(* Logix 5000 AddOnInstructionDefinition export Banner_Q2X_Param_v4; software revision 33.00; part 2 of 3 *)
(* tags used below, declared in another part *)
   Q2X : Banner_Q2X_v4;
   Port_Data : Banner_IOL_Port_v4;
   Port : DINT;
   Local_Control : DINT;
   Command_Being_Processed : BOOL;
   Update_Archive : BOOL;
   Index_Write_Inprocess : INT;
   Index_Write_Control : INT;
   Inprocess_Index : DINT;
(* Banner_Q2X_Param_v4, continued *)

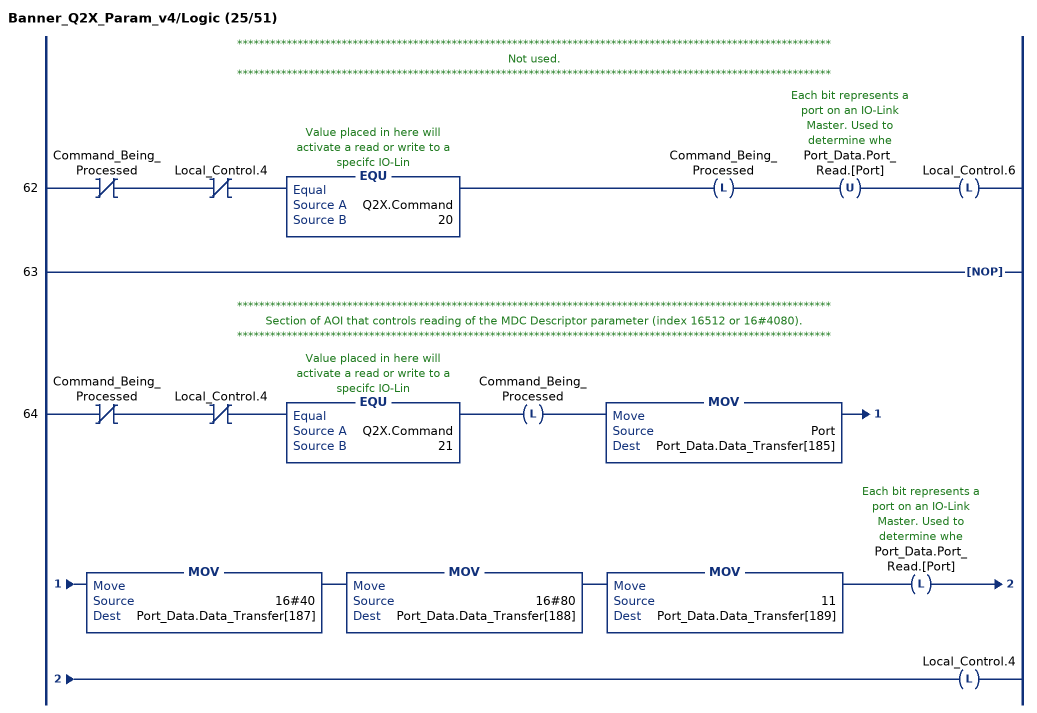
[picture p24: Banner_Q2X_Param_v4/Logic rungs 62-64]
   // ************************************************************************************************************
   // Not used.
   // ************************************************************************************************************
   62: XIO(Command_Being_Processed)XIO(Local_Control.4)EQU(Q2X.Command,20)OTL(Command_Being_Processed)OTU(Port_Data.Port_Read.[Port])OTL(Local_Control.6);
   63: NOP();
   // ************************************************************************************************************
   // Section of AOI that controls reading of the MDC Descriptor parameter (index 16512 or 16#4080).
   // ************************************************************************************************************
   64: XIO(Command_Being_Processed)XIO(Local_Control.4)EQU(Q2X.Command,21)OTL(Command_Being_Processed)MOV(Port,Port_Data.Data_Transfer[185])MOV(16#40,Port_Data.Data_Transfer[187])MOV(16#80,Port_Data.Data_Transfer[188])MOV(11,Port_Data.Data_Transfer[189])OTL(Port_Data.Port_Read.[Port])OTL(Local_Control.4);
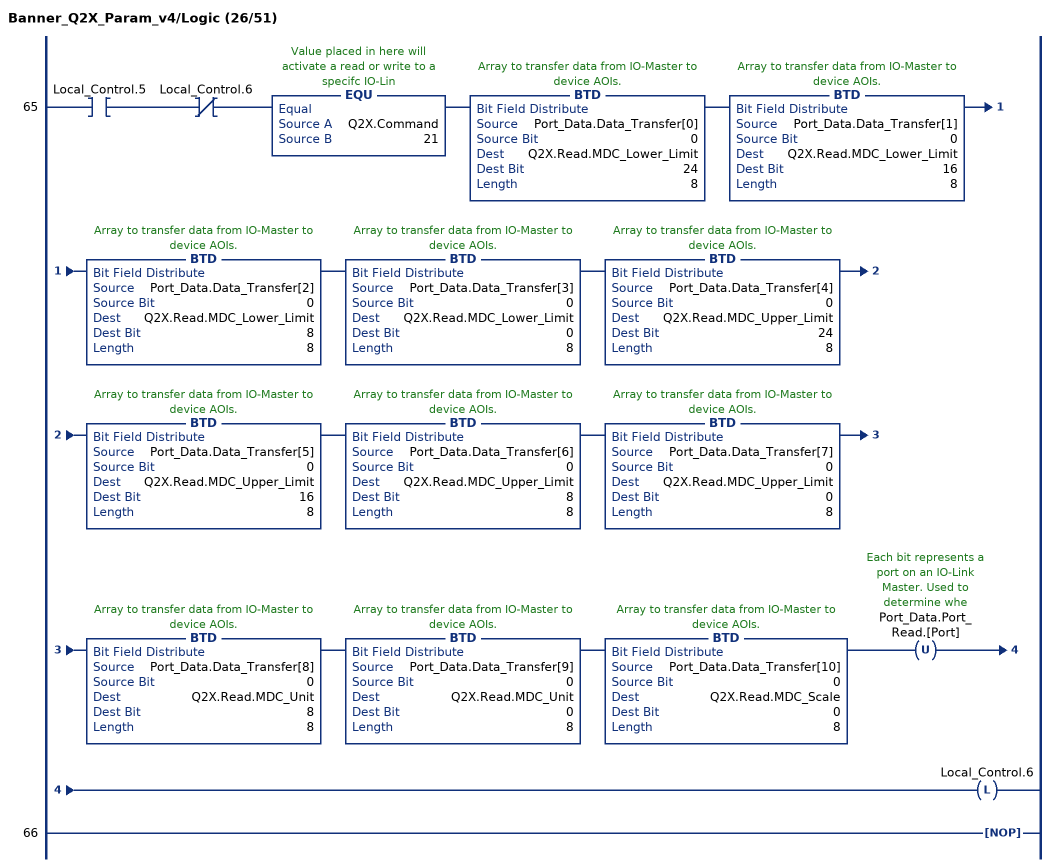
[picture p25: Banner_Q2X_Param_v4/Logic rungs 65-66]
   65: XIC(Local_Control.5)XIO(Local_Control.6)EQU(Q2X.Command,21)BTD(Port_Data.Data_Transfer[0],0,Q2X.Read.MDC_Lower_Limit,24,8)BTD(Port_Data.Data_Transfer[1],0,Q2X.Read.MDC_Lower_Limit,16,8)BTD(Port_Data.Data_Transfer[2],0,Q2X.Read.MDC_Lower_Limit,8,8)BTD(Port_Data.Data_Transfer[3],0,Q2X.Read.MDC_Lower_Limit,0,8)BTD(Port_Data.Data_Transfer[4],0,Q2X.Read.MDC_Upper_Limit,24,8)BTD(Port_Data.Data_Transfer[5],0,Q2X.Read.MDC_Upper_Limit,16,8)BTD(Port_Data.Data_Transfer[6],0,Q2X.Read.MDC_Upper_Limit,8,8)BTD(Port_Data.Data_Transfer[7],0,Q2X.Read.MDC_Upper_Limit,0,8)BTD(Port_Data.Data_Transfer[8],0,Q2X.Read.MDC_Unit,8,8)BTD(Port_Data.Data_Transfer[9],0,Q2X.Read.MDC_Unit,0,8)BTD(Port_Data.Data_Transfer[10],0,Q2X.Read.MDC_Scale,0,8)OTU(Port_Data.Port_Read.[Port])OTL(Local_Control.6);
   66: NOP();
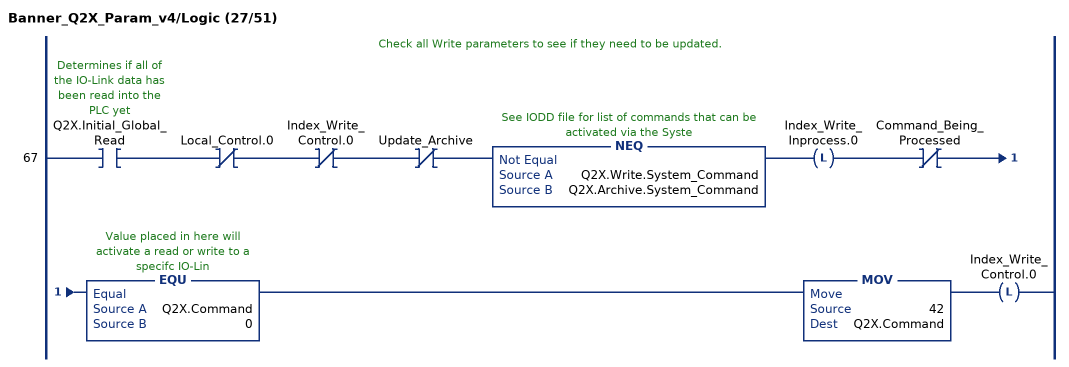
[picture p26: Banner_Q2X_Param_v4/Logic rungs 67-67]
   // Check all Write parameters to see if they need to be updated.
   67: XIC(Q2X.Initial_Global_Read)XIO(Local_Control.0)XIO(Index_Write_Control.0)XIO(Update_Archive)NEQ(Q2X.Write.System_Command,Q2X.Archive.System_Command)OTL(Index_Write_Inprocess.0)XIO(Command_Being_Processed)EQU(Q2X.Command,0)MOV(42,Q2X.Command)OTL(Index_Write_Control.0);
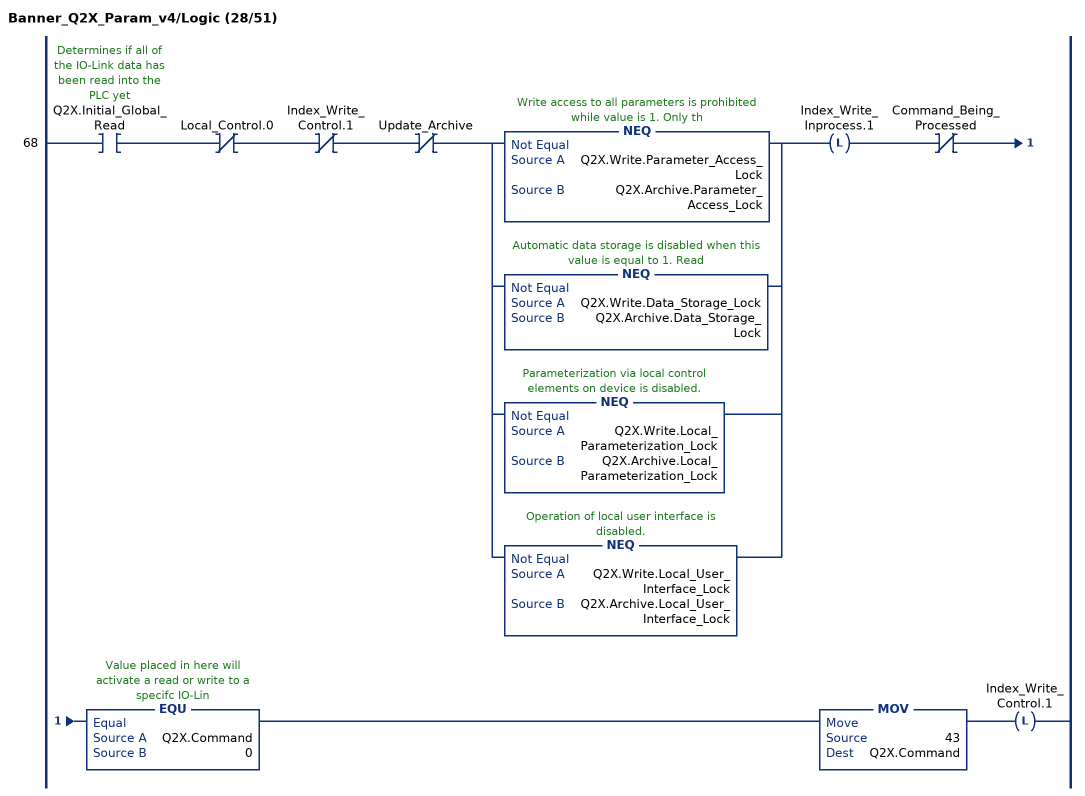
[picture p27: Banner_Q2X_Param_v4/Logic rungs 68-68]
   68: XIC(Q2X.Initial_Global_Read)XIO(Local_Control.0)XIO(Index_Write_Control.1)XIO(Update_Archive)[NEQ(Q2X.Write.Parameter_Access_Lock,Q2X.Archive.Parameter_Access_Lock) ,NEQ(Q2X.Write.Data_Storage_Lock,Q2X.Archive.Data_Storage_Lock) ,NEQ(Q2X.Write.Local_Parameterization_Lock,Q2X.Archive.Local_Parameterization_Lock) ,NEQ(Q2X.Write.Local_User_Interface_Lock,Q2X.Archive.Local_User_Interface_Lock) ]OTL(Index_Write_Inprocess.1)XIO(Command_Being_Processed)EQU(Q2X.Command,0)MOV(43,Q2X.Command)OTL(Index_Write_Control.1);
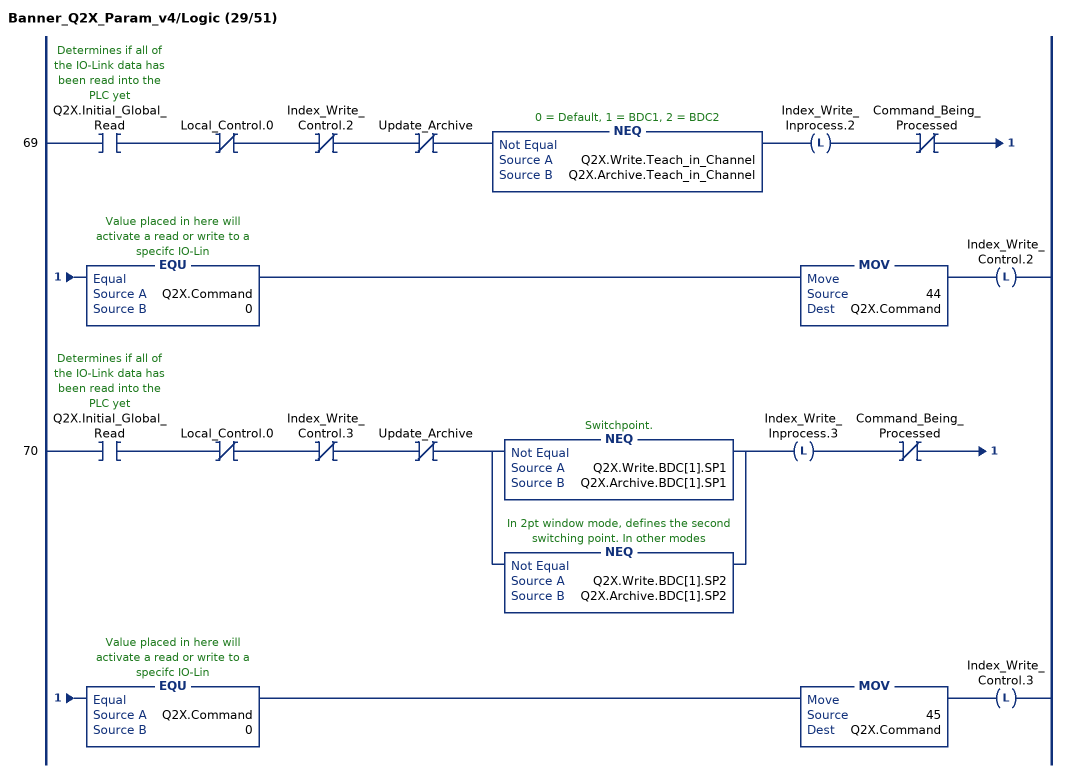
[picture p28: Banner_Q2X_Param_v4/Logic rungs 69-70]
   69: XIC(Q2X.Initial_Global_Read)XIO(Local_Control.0)XIO(Index_Write_Control.2)XIO(Update_Archive)NEQ(Q2X.Write.Teach_in_Channel,Q2X.Archive.Teach_in_Channel)OTL(Index_Write_Inprocess.2)XIO(Command_Being_Processed)EQU(Q2X.Command,0)MOV(44,Q2X.Command)OTL(Index_Write_Control.2);
   70: XIC(Q2X.Initial_Global_Read)XIO(Local_Control.0)XIO(Index_Write_Control.3)XIO(Update_Archive)[NEQ(Q2X.Write.BDC[1].SP1,Q2X.Archive.BDC[1].SP1) ,NEQ(Q2X.Write.BDC[1].SP2,Q2X.Archive.BDC[1].SP2) ]OTL(Index_Write_Inprocess.3)XIO(Command_Being_Processed)EQU(Q2X.Command,0)MOV(45,Q2X.Command)OTL(Index_Write_Control.3);
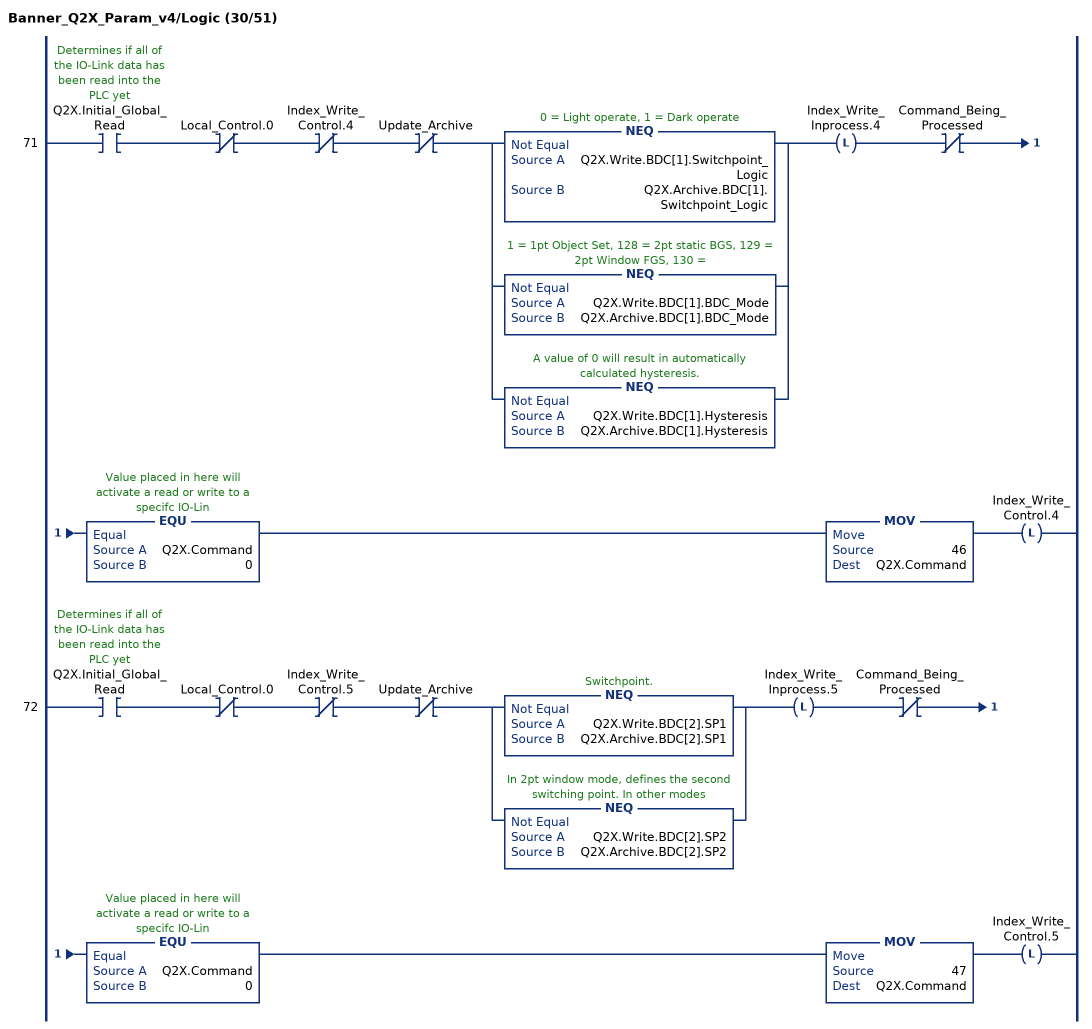
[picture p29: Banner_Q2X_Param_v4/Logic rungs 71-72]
   71: XIC(Q2X.Initial_Global_Read)XIO(Local_Control.0)XIO(Index_Write_Control.4)XIO(Update_Archive)[NEQ(Q2X.Write.BDC[1].Switchpoint_Logic,Q2X.Archive.BDC[1].Switchpoint_Logic) ,NEQ(Q2X.Write.BDC[1].BDC_Mode,Q2X.Archive.BDC[1].BDC_Mode) ,NEQ(Q2X.Write.BDC[1].Hysteresis,Q2X.Archive.BDC[1].Hysteresis) ]OTL(Index_Write_Inprocess.4)XIO(Command_Being_Processed)EQU(Q2X.Command,0)MOV(46,Q2X.Command)OTL(Index_Write_Control.4);
   72: XIC(Q2X.Initial_Global_Read)XIO(Local_Control.0)XIO(Index_Write_Control.5)XIO(Update_Archive)[NEQ(Q2X.Write.BDC[2].SP1,Q2X.Archive.BDC[2].SP1) ,NEQ(Q2X.Write.BDC[2].SP2,Q2X.Archive.BDC[2].SP2) ]OTL(Index_Write_Inprocess.5)XIO(Command_Being_Processed)EQU(Q2X.Command,0)MOV(47,Q2X.Command)OTL(Index_Write_Control.5);
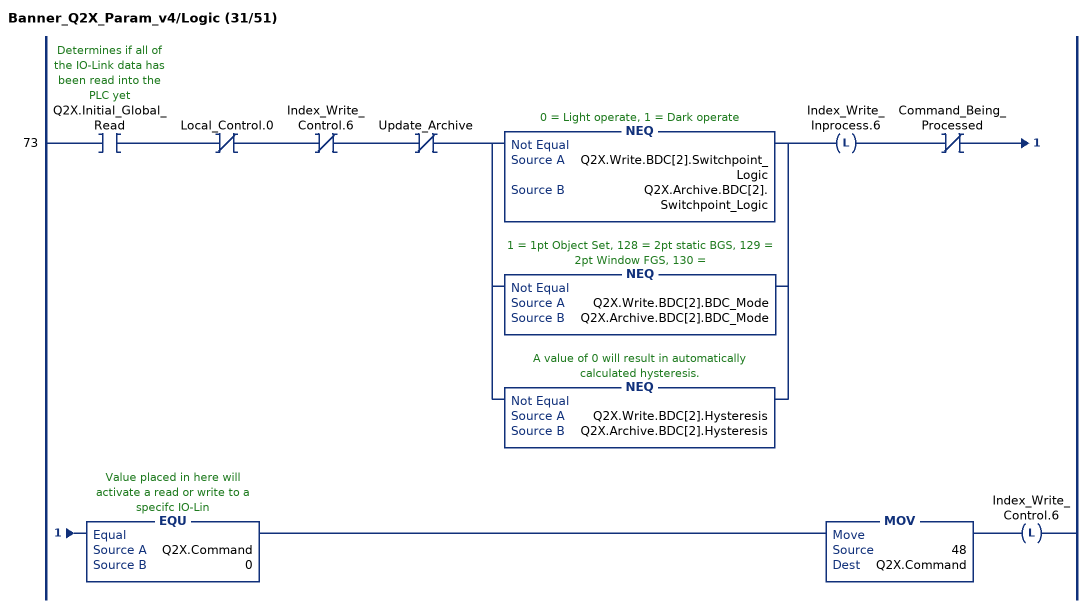
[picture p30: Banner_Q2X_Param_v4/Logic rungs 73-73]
   73: XIC(Q2X.Initial_Global_Read)XIO(Local_Control.0)XIO(Index_Write_Control.6)XIO(Update_Archive)[NEQ(Q2X.Write.BDC[2].Switchpoint_Logic,Q2X.Archive.BDC[2].Switchpoint_Logic) ,NEQ(Q2X.Write.BDC[2].BDC_Mode,Q2X.Archive.BDC[2].BDC_Mode) ,NEQ(Q2X.Write.BDC[2].Hysteresis,Q2X.Archive.BDC[2].Hysteresis) ]OTL(Index_Write_Inprocess.6)XIO(Command_Being_Processed)EQU(Q2X.Command,0)MOV(48,Q2X.Command)OTL(Index_Write_Control.6);
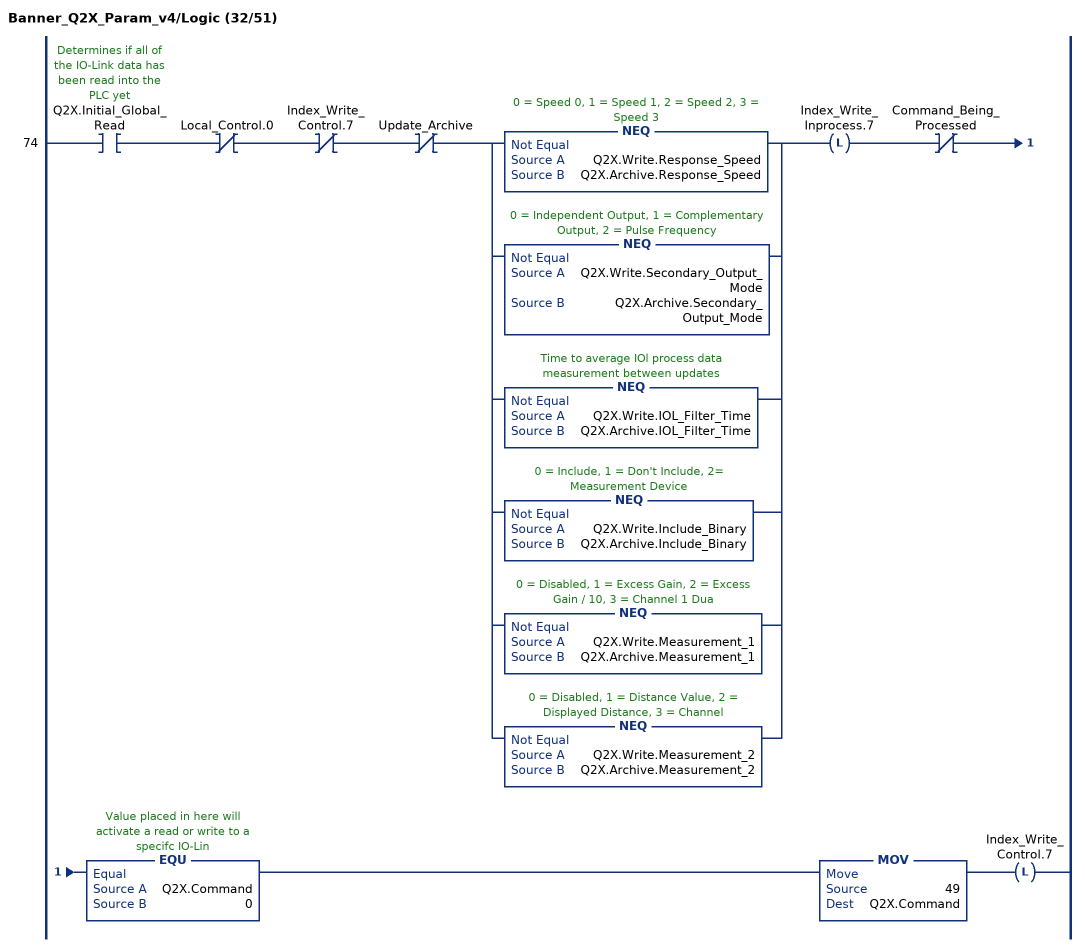
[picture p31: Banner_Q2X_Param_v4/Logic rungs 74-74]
   74: XIC(Q2X.Initial_Global_Read)XIO(Local_Control.0)XIO(Index_Write_Control.7)XIO(Update_Archive)[NEQ(Q2X.Write.Response_Speed,Q2X.Archive.Response_Speed) ,NEQ(Q2X.Write.Secondary_Output_Mode,Q2X.Archive.Secondary_Output_Mode) ,NEQ(Q2X.Write.IOL_Filter_Time,Q2X.Archive.IOL_Filter_Time) ,NEQ(Q2X.Write.Include_Binary,Q2X.Archive.Include_Binary) ,NEQ(Q2X.Write.Measurement_1,Q2X.Archive.Measurement_1) ,NEQ(Q2X.Write.Measurement_2,Q2X.Archive.Measurement_2) ]OTL(Index_Write_Inprocess.7)XIO(Command_Being_Processed)EQU(Q2X.Command,0)MOV(49,Q2X.Command)OTL(Index_Write_Control.7);
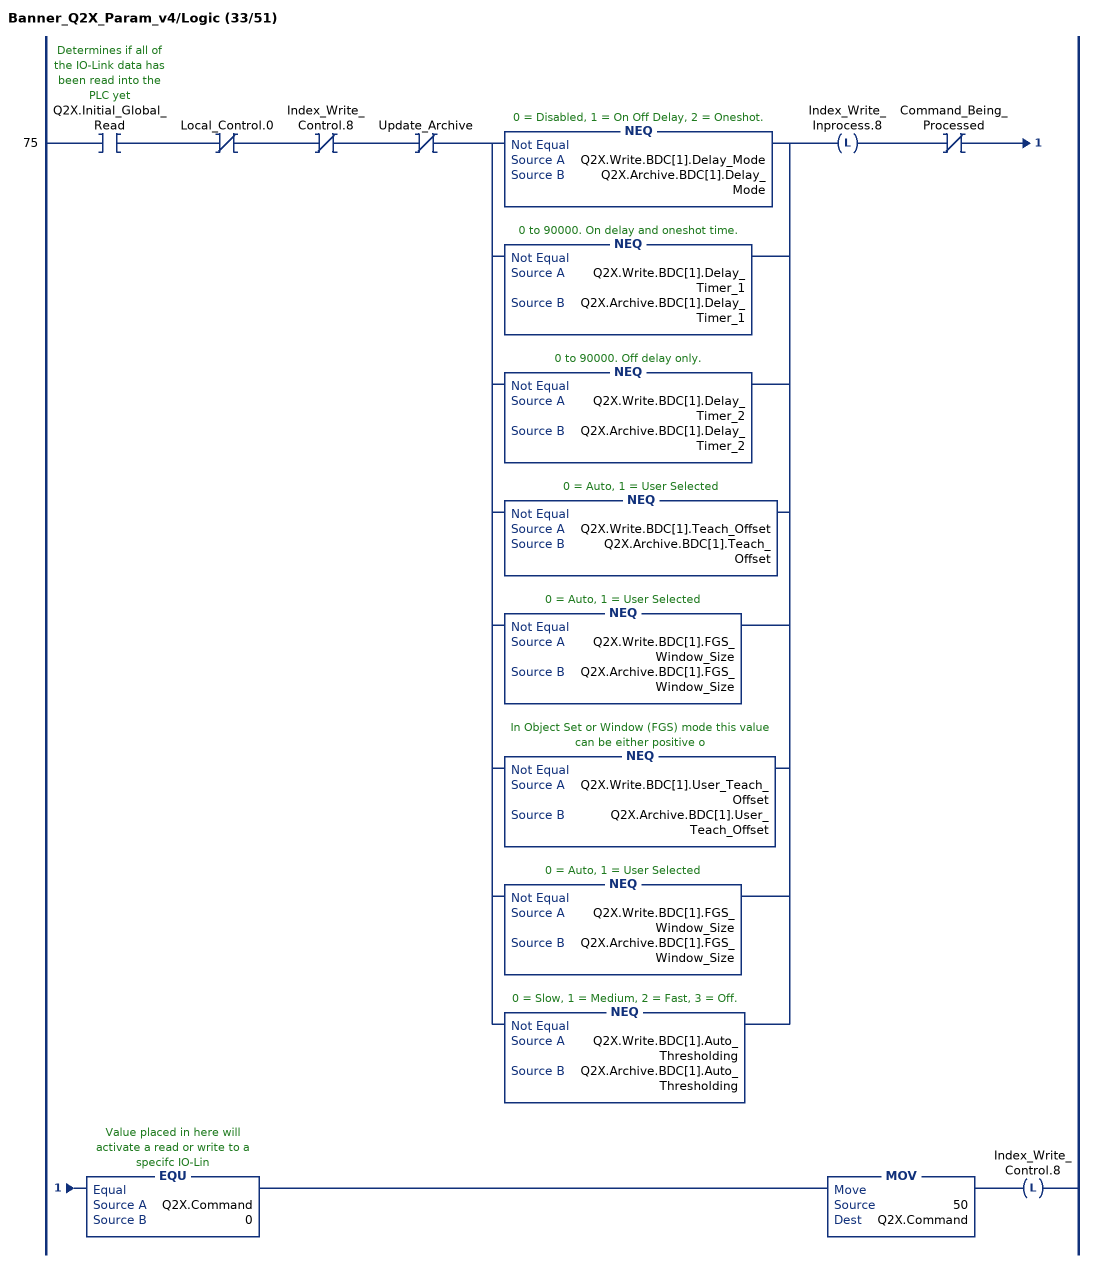
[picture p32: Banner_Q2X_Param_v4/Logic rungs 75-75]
   75: XIC(Q2X.Initial_Global_Read)XIO(Local_Control.0)XIO(Index_Write_Control.8)XIO(Update_Archive)[NEQ(Q2X.Write.BDC[1].Delay_Mode,Q2X.Archive.BDC[1].Delay_Mode) ,NEQ(Q2X.Write.BDC[1].Delay_Timer_1,Q2X.Archive.BDC[1].Delay_Timer_1) ,NEQ(Q2X.Write.BDC[1].Delay_Timer_2,Q2X.Archive.BDC[1].Delay_Timer_2) ,NEQ(Q2X.Write.BDC[1].Teach_Offset,Q2X.Archive.BDC[1].Teach_Offset) ,NEQ(Q2X.Write.BDC[1].FGS_Window_Size,Q2X.Archive.BDC[1].FGS_Window_Size) ,NEQ(Q2X.Write.BDC[1].User_Teach_Offset,Q2X.Archive.BDC[1].User_Teach_Offset) ,NEQ(Q2X.Write.BDC[1].FGS_Window_Size,Q2X.Archive.BDC[1].FGS_Window_Size) ,NEQ(Q2X.Write.BDC[1].Auto_Thresholding,Q2X.Archive.BDC[1].Auto_Thresholding) ]OTL(Index_Write_Inprocess.8)XIO(Command_Being_Processed)EQU(Q2X.Command,0)MOV(50,Q2X.Command)OTL(Index_Write_Control.8);
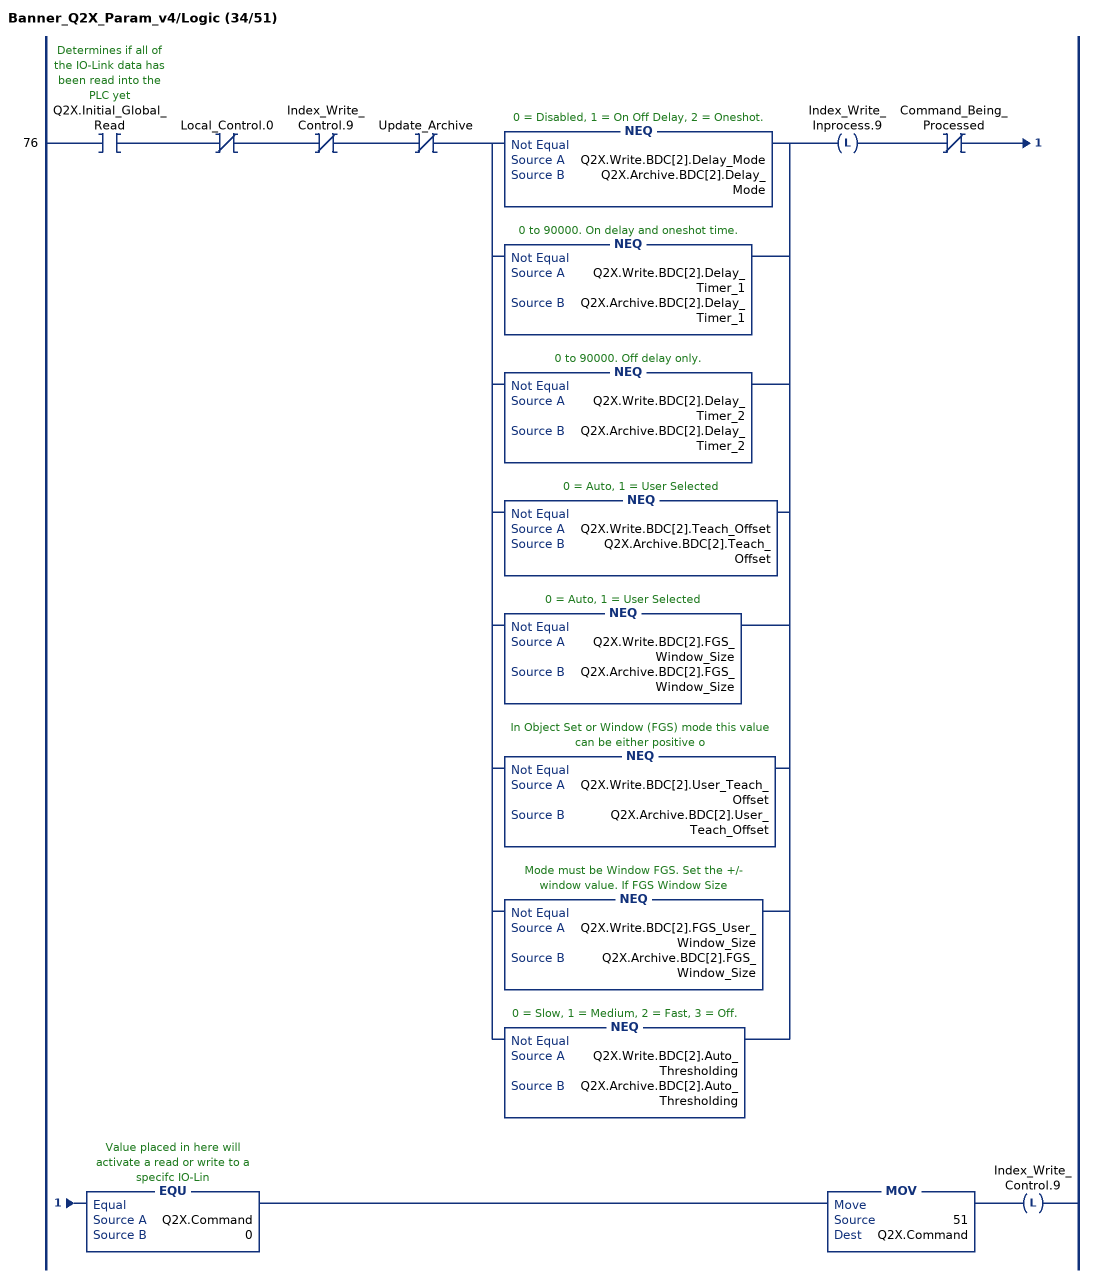
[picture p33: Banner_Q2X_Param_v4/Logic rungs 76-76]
   76: XIC(Q2X.Initial_Global_Read)XIO(Local_Control.0)XIO(Index_Write_Control.9)XIO(Update_Archive)[NEQ(Q2X.Write.BDC[2].Delay_Mode,Q2X.Archive.BDC[2].Delay_Mode) ,NEQ(Q2X.Write.BDC[2].Delay_Timer_1,Q2X.Archive.BDC[2].Delay_Timer_1) ,NEQ(Q2X.Write.BDC[2].Delay_Timer_2,Q2X.Archive.BDC[2].Delay_Timer_2) ,NEQ(Q2X.Write.BDC[2].Teach_Offset,Q2X.Archive.BDC[2].Teach_Offset) ,NEQ(Q2X.Write.BDC[2].FGS_Window_Size,Q2X.Archive.BDC[2].FGS_Window_Size) ,NEQ(Q2X.Write.BDC[2].User_Teach_Offset,Q2X.Archive.BDC[2].User_Teach_Offset) ,NEQ(Q2X.Write.BDC[2].FGS_User_Window_Size,Q2X.Archive.BDC[2].FGS_Window_Size) ,NEQ(Q2X.Write.BDC[2].Auto_Thresholding,Q2X.Archive.BDC[2].Auto_Thresholding) ]OTL(Index_Write_Inprocess.9)XIO(Command_Being_Processed)EQU(Q2X.Command,0)MOV(51,Q2X.Command)OTL(Index_Write_Control.9);
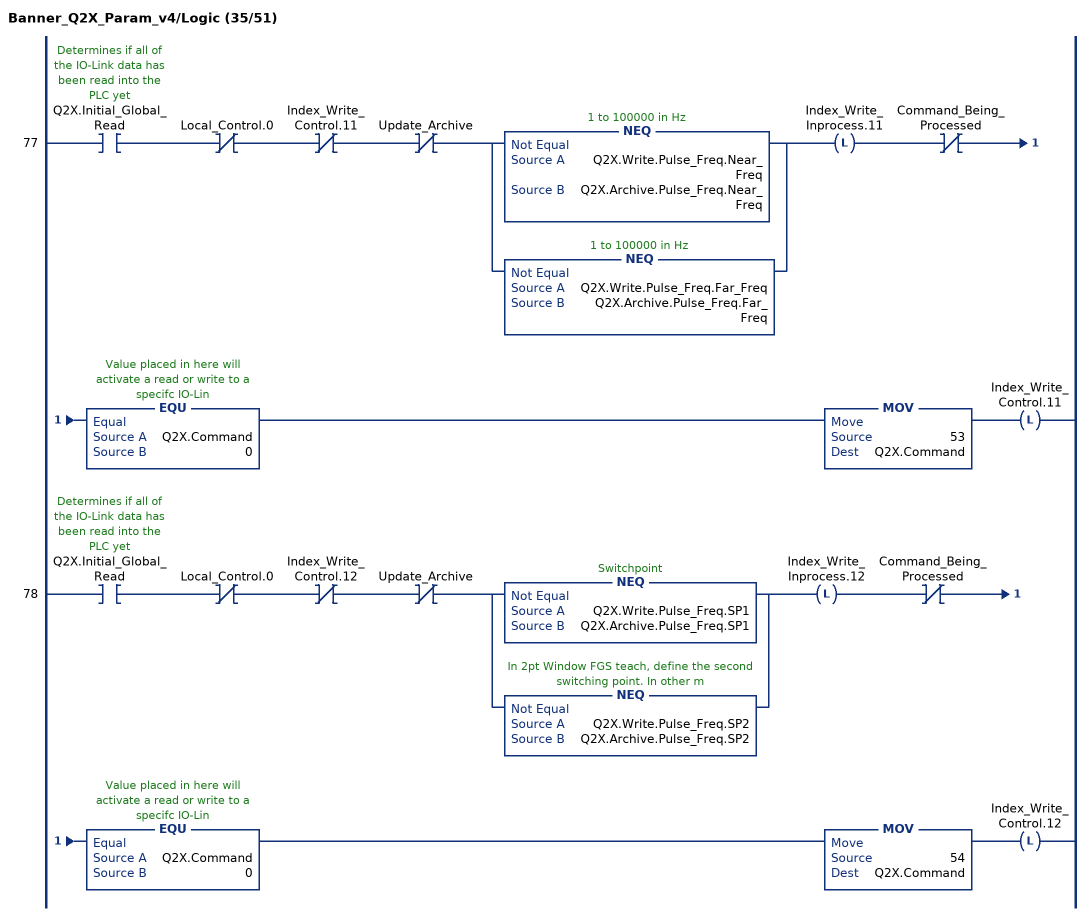
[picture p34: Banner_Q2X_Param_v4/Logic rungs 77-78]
   77: XIC(Q2X.Initial_Global_Read)XIO(Local_Control.0)XIO(Index_Write_Control.11)XIO(Update_Archive)[NEQ(Q2X.Write.Pulse_Freq.Near_Freq,Q2X.Archive.Pulse_Freq.Near_Freq) ,NEQ(Q2X.Write.Pulse_Freq.Far_Freq,Q2X.Archive.Pulse_Freq.Far_Freq) ]OTL(Index_Write_Inprocess.11)XIO(Command_Being_Processed)EQU(Q2X.Command,0)MOV(53,Q2X.Command)OTL(Index_Write_Control.11);
   78: XIC(Q2X.Initial_Global_Read)XIO(Local_Control.0)XIO(Index_Write_Control.12)XIO(Update_Archive)[NEQ(Q2X.Write.Pulse_Freq.SP1,Q2X.Archive.Pulse_Freq.SP1) ,NEQ(Q2X.Write.Pulse_Freq.SP2,Q2X.Archive.Pulse_Freq.SP2) ]OTL(Index_Write_Inprocess.12)XIO(Command_Being_Processed)EQU(Q2X.Command,0)MOV(54,Q2X.Command)OTL(Index_Write_Control.12);
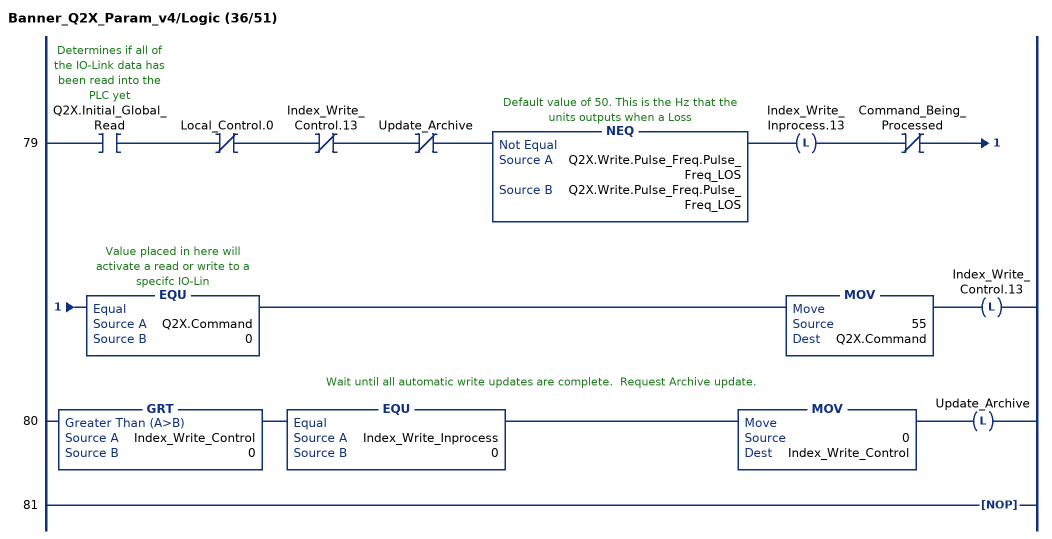
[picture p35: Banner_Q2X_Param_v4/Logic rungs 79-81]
   79: XIC(Q2X.Initial_Global_Read)XIO(Local_Control.0)XIO(Index_Write_Control.13)XIO(Update_Archive)NEQ(Q2X.Write.Pulse_Freq.Pulse_Freq_LOS,Q2X.Write.Pulse_Freq.Pulse_Freq_LOS)OTL(Index_Write_Inprocess.13)XIO(Command_Being_Processed)EQU(Q2X.Command,0)MOV(55,Q2X.Command)OTL(Index_Write_Control.13);
   // Wait until all automatic write updates are complete.  Request Archive update.
   80: GRT(Index_Write_Control,0)EQU(Index_Write_Inprocess,0)MOV(0,Index_Write_Control)OTL(Update_Archive);
   81: NOP();
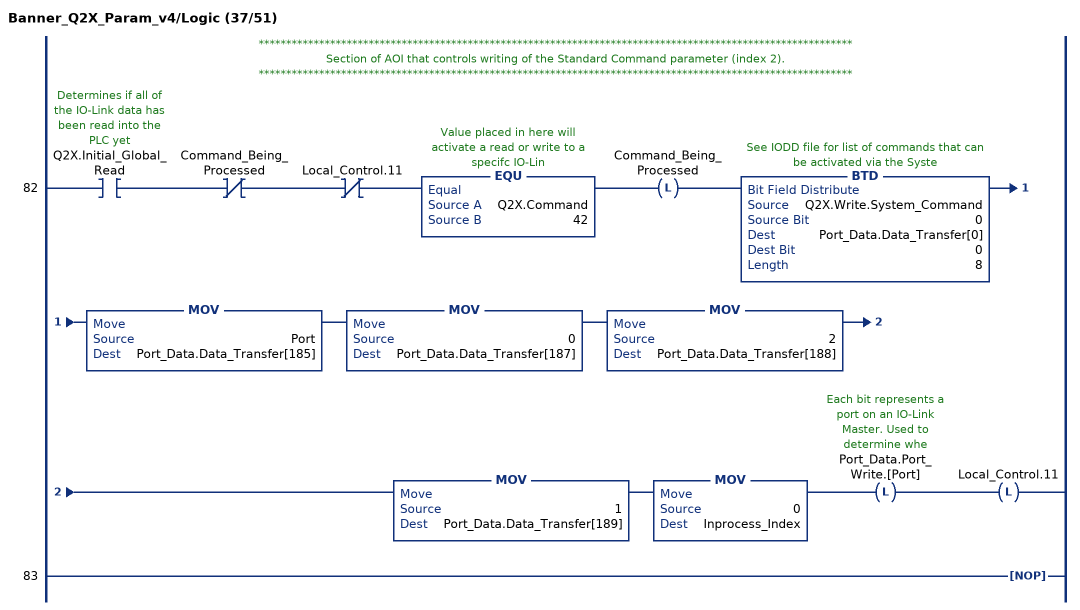
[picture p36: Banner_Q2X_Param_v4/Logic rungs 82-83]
   // ************************************************************************************************************
   // Section of AOI that controls writing of the Standard Command parameter (index 2).
   // ************************************************************************************************************
   82: XIC(Q2X.Initial_Global_Read)XIO(Command_Being_Processed)XIO(Local_Control.11)EQU(Q2X.Command,42)OTL(Command_Being_Processed)BTD(Q2X.Write.System_Command,0,Port_Data.Data_Transfer[0],0,8)MOV(Port,Port_Data.Data_Transfer[185])MOV(0,Port_Data.Data_Transfer[187])MOV(2,Port_Data.Data_Transfer[188])MOV(1,Port_Data.Data_Transfer[189])MOV(0,Inprocess_Index)OTL(Port_Data.Port_Write.[Port])OTL(Local_Control.11);
   83: NOP();
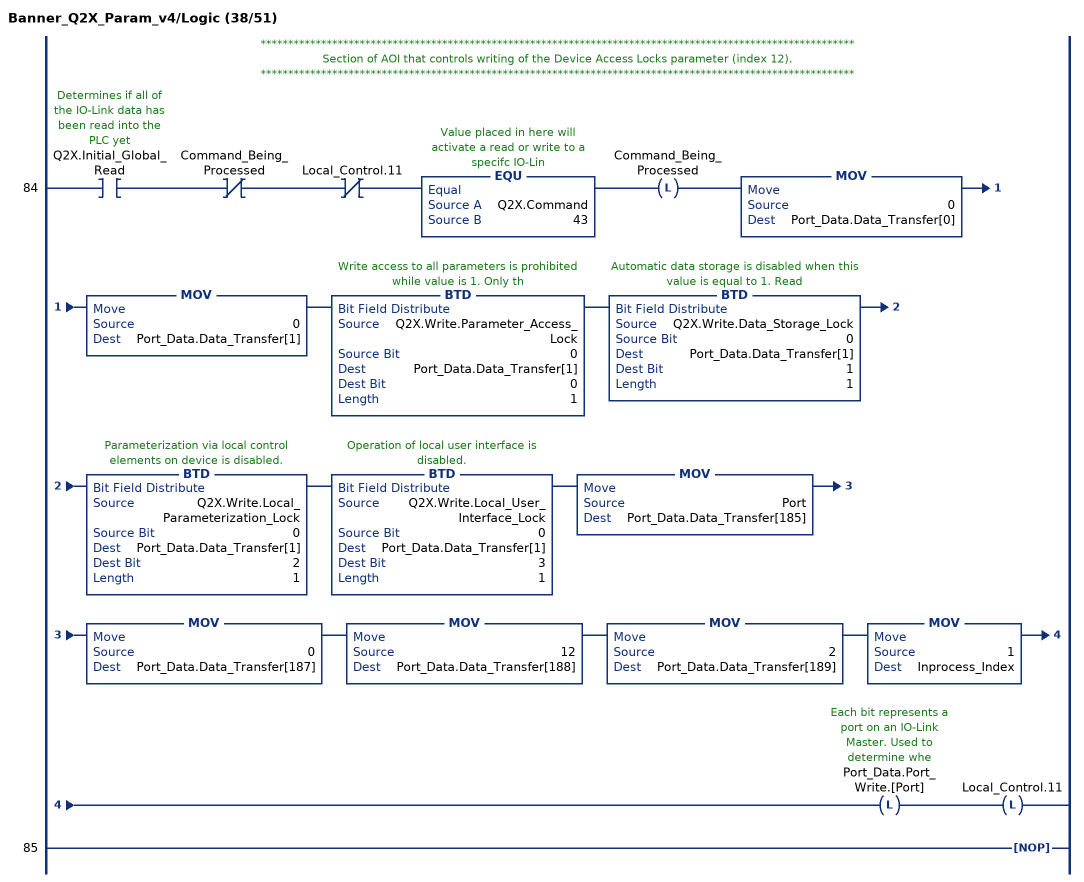
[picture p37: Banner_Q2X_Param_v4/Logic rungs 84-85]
   // ************************************************************************************************************
   // Section of AOI that controls writing of the Device Access Locks parameter (index 12).
   // ************************************************************************************************************
   84: XIC(Q2X.Initial_Global_Read)XIO(Command_Being_Processed)XIO(Local_Control.11)EQU(Q2X.Command,43)OTL(Command_Being_Processed)MOV(0,Port_Data.Data_Transfer[0])MOV(0,Port_Data.Data_Transfer[1])BTD(Q2X.Write.Parameter_Access_Lock,0,Port_Data.Data_Transfer[1],0,1)BTD(Q2X.Write.Data_Storage_Lock,0,Port_Data.Data_Transfer[1],1,1)BTD(Q2X.Write.Local_Parameterization_Lock,0,Port_Data.Data_Transfer[1],2,1)BTD(Q2X.Write.Local_User_Interface_Lock,0,Port_Data.Data_Transfer[1],3,1)MOV(Port,Port_Data.Data_Transfer[185])MOV(0,Port_Data.Data_Transfer[187])MOV(12,Port_Data.Data_Transfer[188])MOV(2,Port_Data.Data_Transfer[189])MOV(1,Inprocess_Index)OTL(Port_Data.Port_Write.[Port])OTL(Local_Control.11);
   85: NOP();
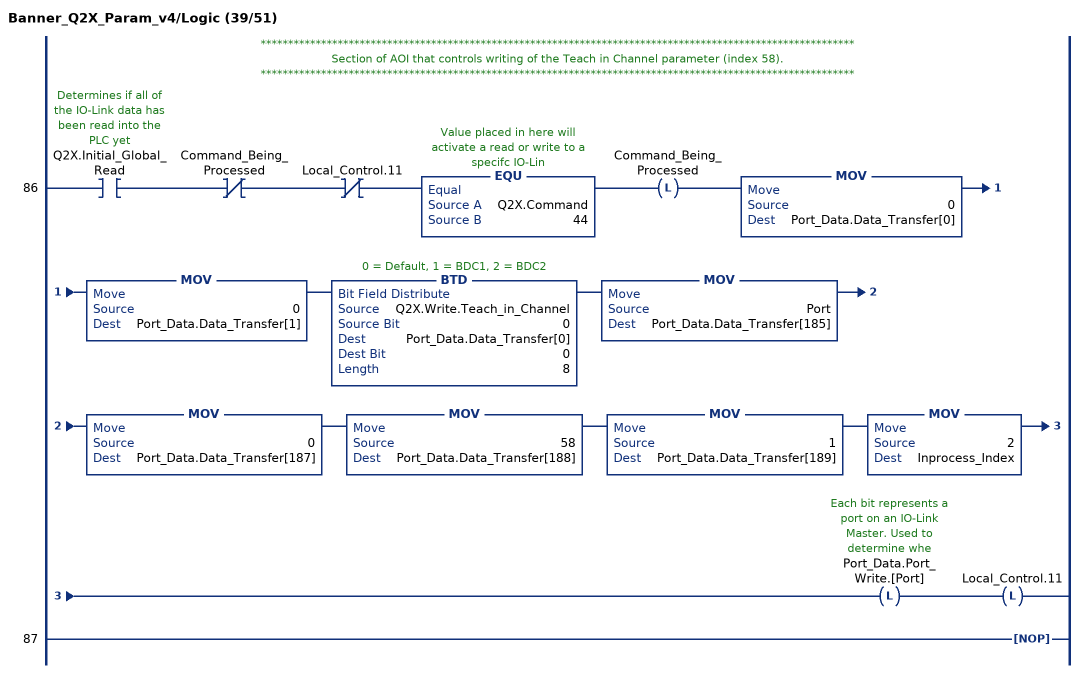
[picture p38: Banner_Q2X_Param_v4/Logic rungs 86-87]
   // ************************************************************************************************************
   // Section of AOI that controls writing of the Teach in Channel parameter (index 58).
   // ************************************************************************************************************
   86: XIC(Q2X.Initial_Global_Read)XIO(Command_Being_Processed)XIO(Local_Control.11)EQU(Q2X.Command,44)OTL(Command_Being_Processed)MOV(0,Port_Data.Data_Transfer[0])MOV(0,Port_Data.Data_Transfer[1])BTD(Q2X.Write.Teach_in_Channel,0,Port_Data.Data_Transfer[0],0,8)MOV(Port,Port_Data.Data_Transfer[185])MOV(0,Port_Data.Data_Transfer[187])MOV(58,Port_Data.Data_Transfer[188])MOV(1,Port_Data.Data_Transfer[189])MOV(2,Inprocess_Index)OTL(Port_Data.Port_Write.[Port])OTL(Local_Control.11);
   87: NOP();
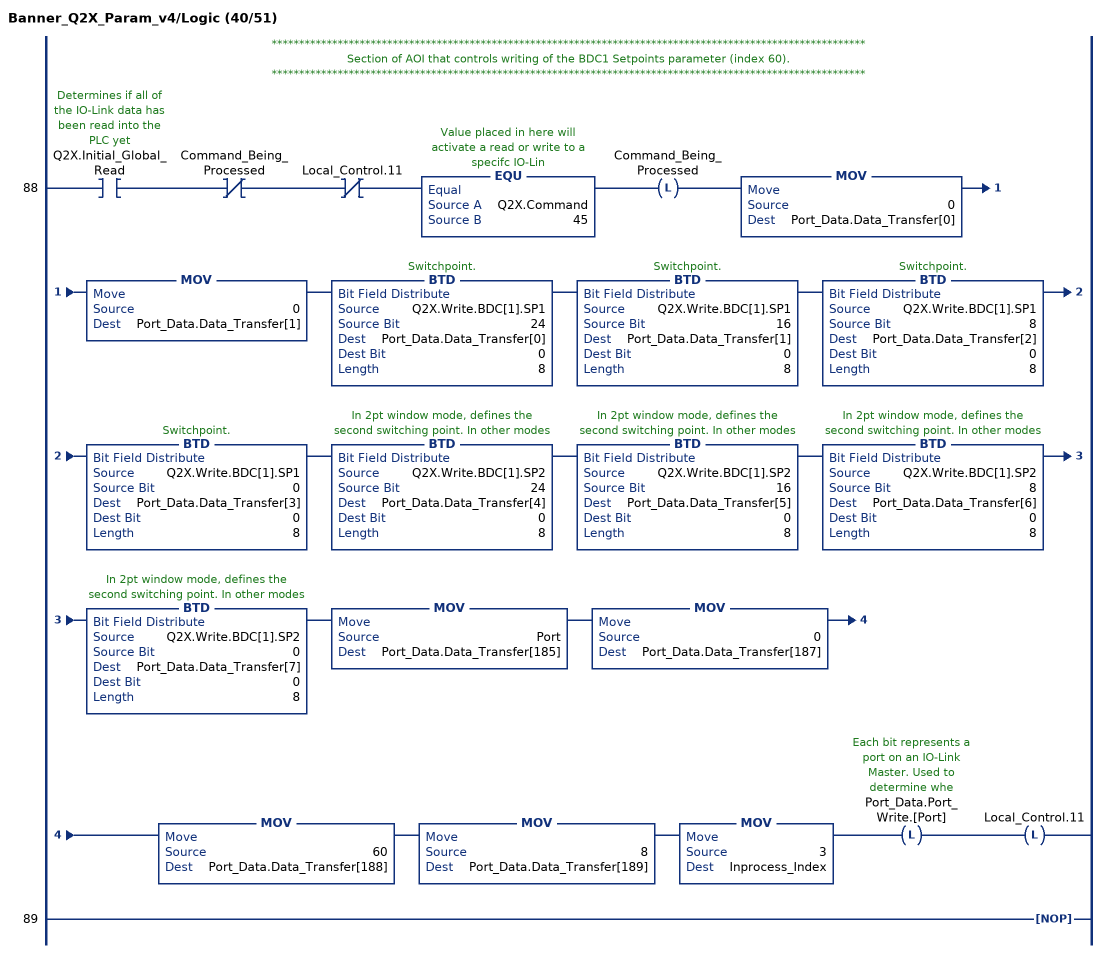
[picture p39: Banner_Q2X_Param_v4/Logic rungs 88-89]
   // ************************************************************************************************************
   // Section of AOI that controls writing of the BDC1 Setpoints parameter (index 60).
   // ************************************************************************************************************
   88: XIC(Q2X.Initial_Global_Read)XIO(Command_Being_Processed)XIO(Local_Control.11)EQU(Q2X.Command,45)OTL(Command_Being_Processed)MOV(0,Port_Data.Data_Transfer[0])MOV(0,Port_Data.Data_Transfer[1])BTD(Q2X.Write.BDC[1].SP1,24,Port_Data.Data_Transfer[0],0,8)BTD(Q2X.Write.BDC[1].SP1,16,Port_Data.Data_Transfer[1],0,8)BTD(Q2X.Write.BDC[1].SP1,8,Port_Data.Data_Transfer[2],0,8)BTD(Q2X.Write.BDC[1].SP1,0,Port_Data.Data_Transfer[3],0,8)BTD(Q2X.Write.BDC[1].SP2,24,Port_Data.Data_Transfer[4],0,8)BTD(Q2X.Write.BDC[1].SP2,16,Port_Data.Data_Transfer[5],0,8)BTD(Q2X.Write.BDC[1].SP2,8,Port_Data.Data_Transfer[6],0,8)BTD(Q2X.Write.BDC[1].SP2,0,Port_Data.Data_Transfer[7],0,8)MOV(Port,Port_Data.Data_Transfer[185])MOV(0,Port_Data.Data_Transfer[187])MOV(60,Port_Data.Data_Transfer[188])MOV(8,Port_Data.Data_Transfer[189])MOV(3,Inprocess_Index)OTL(Port_Data.Port_Write.[Port])OTL(Local_Control.11);
   89: NOP();
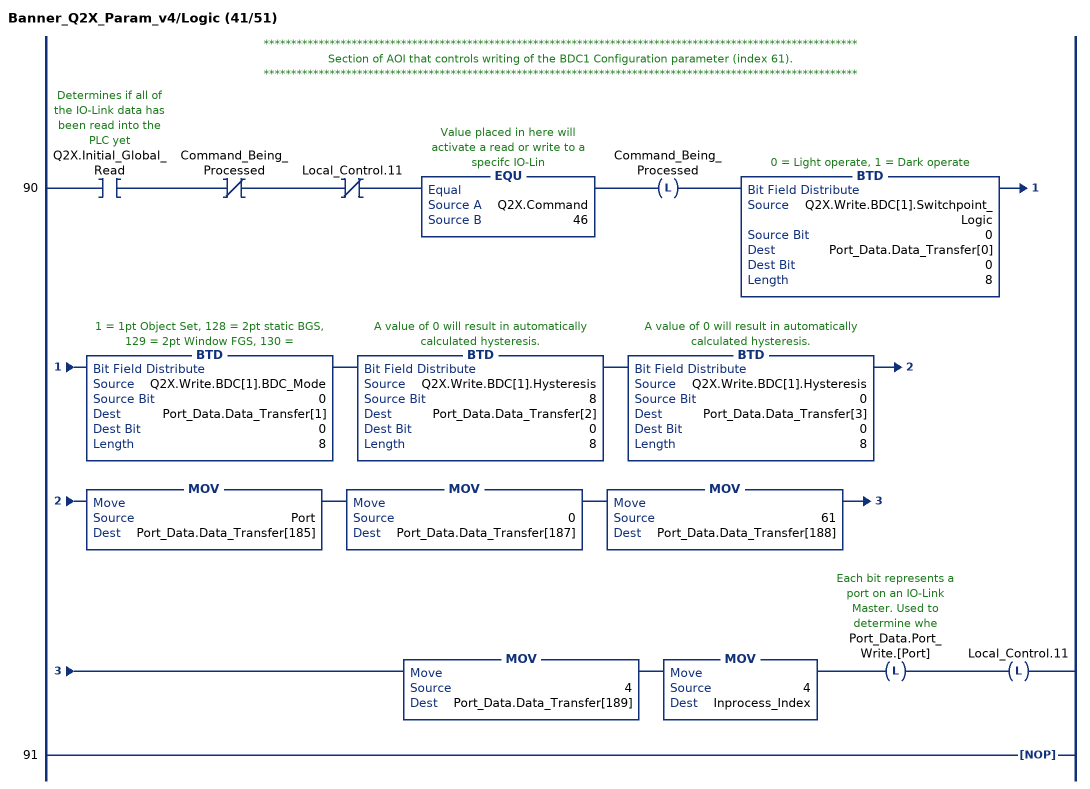
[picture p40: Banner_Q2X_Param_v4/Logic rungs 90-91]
   // ************************************************************************************************************
   // Section of AOI that controls writing of the BDC1 Configuration parameter (index 61).
   // ************************************************************************************************************
   90: XIC(Q2X.Initial_Global_Read)XIO(Command_Being_Processed)XIO(Local_Control.11)EQU(Q2X.Command,46)OTL(Command_Being_Processed)BTD(Q2X.Write.BDC[1].Switchpoint_Logic,0,Port_Data.Data_Transfer[0],0,8)BTD(Q2X.Write.BDC[1].BDC_Mode,0,Port_Data.Data_Transfer[1],0,8)BTD(Q2X.Write.BDC[1].Hysteresis,8,Port_Data.Data_Transfer[2],0,8)BTD(Q2X.Write.BDC[1].Hysteresis,0,Port_Data.Data_Transfer[3],0,8)MOV(Port,Port_Data.Data_Transfer[185])MOV(0,Port_Data.Data_Transfer[187])MOV(61,Port_Data.Data_Transfer[188])MOV(4,Port_Data.Data_Transfer[189])MOV(4,Inprocess_Index)OTL(Port_Data.Port_Write.[Port])OTL(Local_Control.11);
   91: NOP();
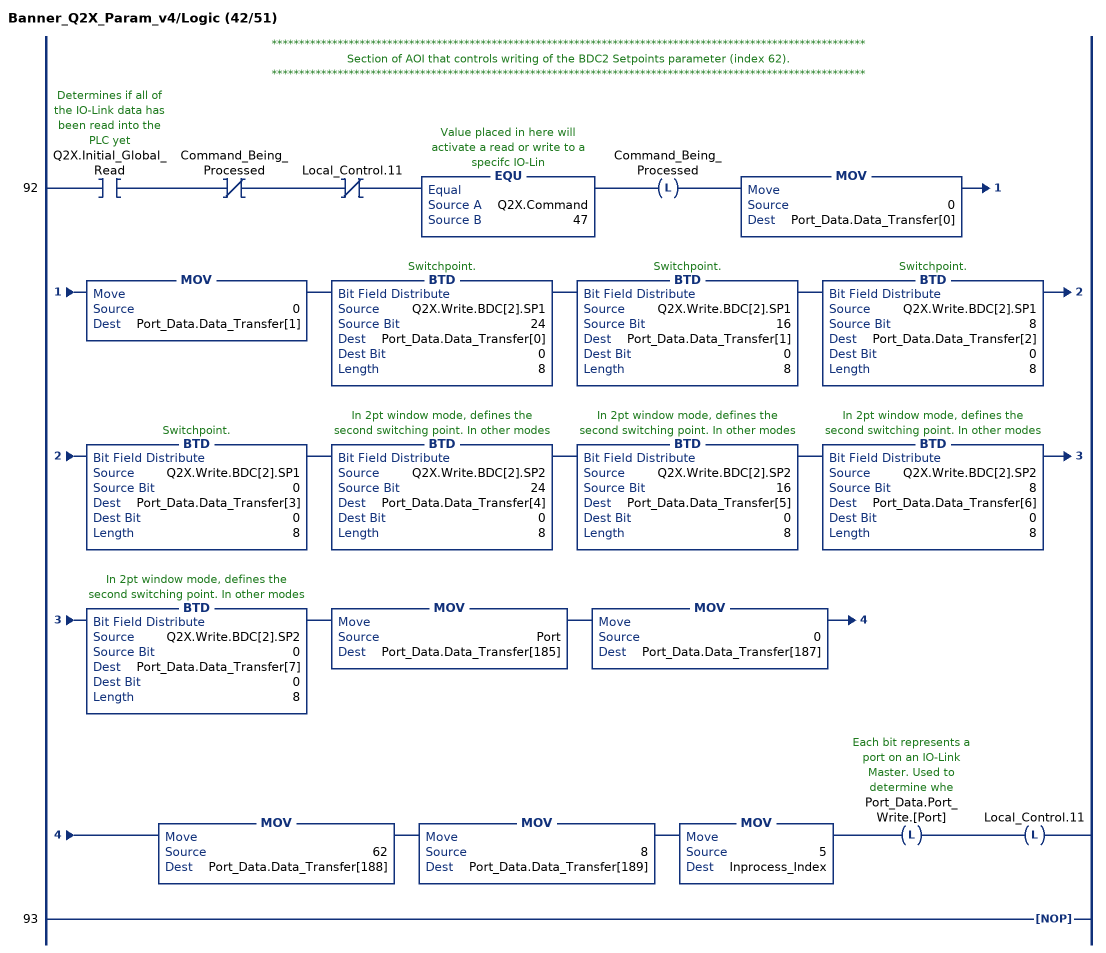
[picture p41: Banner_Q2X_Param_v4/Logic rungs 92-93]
   // ************************************************************************************************************
   // Section of AOI that controls writing of the BDC2 Setpoints parameter (index 62).
   // ************************************************************************************************************
   92: XIC(Q2X.Initial_Global_Read)XIO(Command_Being_Processed)XIO(Local_Control.11)EQU(Q2X.Command,47)OTL(Command_Being_Processed)MOV(0,Port_Data.Data_Transfer[0])MOV(0,Port_Data.Data_Transfer[1])BTD(Q2X.Write.BDC[2].SP1,24,Port_Data.Data_Transfer[0],0,8)BTD(Q2X.Write.BDC[2].SP1,16,Port_Data.Data_Transfer[1],0,8)BTD(Q2X.Write.BDC[2].SP1,8,Port_Data.Data_Transfer[2],0,8)BTD(Q2X.Write.BDC[2].SP1,0,Port_Data.Data_Transfer[3],0,8)BTD(Q2X.Write.BDC[2].SP2,24,Port_Data.Data_Transfer[4],0,8)BTD(Q2X.Write.BDC[2].SP2,16,Port_Data.Data_Transfer[5],0,8)BTD(Q2X.Write.BDC[2].SP2,8,Port_Data.Data_Transfer[6],0,8)BTD(Q2X.Write.BDC[2].SP2,0,Port_Data.Data_Transfer[7],0,8)MOV(Port,Port_Data.Data_Transfer[185])MOV(0,Port_Data.Data_Transfer[187])MOV(62,Port_Data.Data_Transfer[188])MOV(8,Port_Data.Data_Transfer[189])MOV(5,Inprocess_Index)OTL(Port_Data.Port_Write.[Port])OTL(Local_Control.11);
   93: NOP();
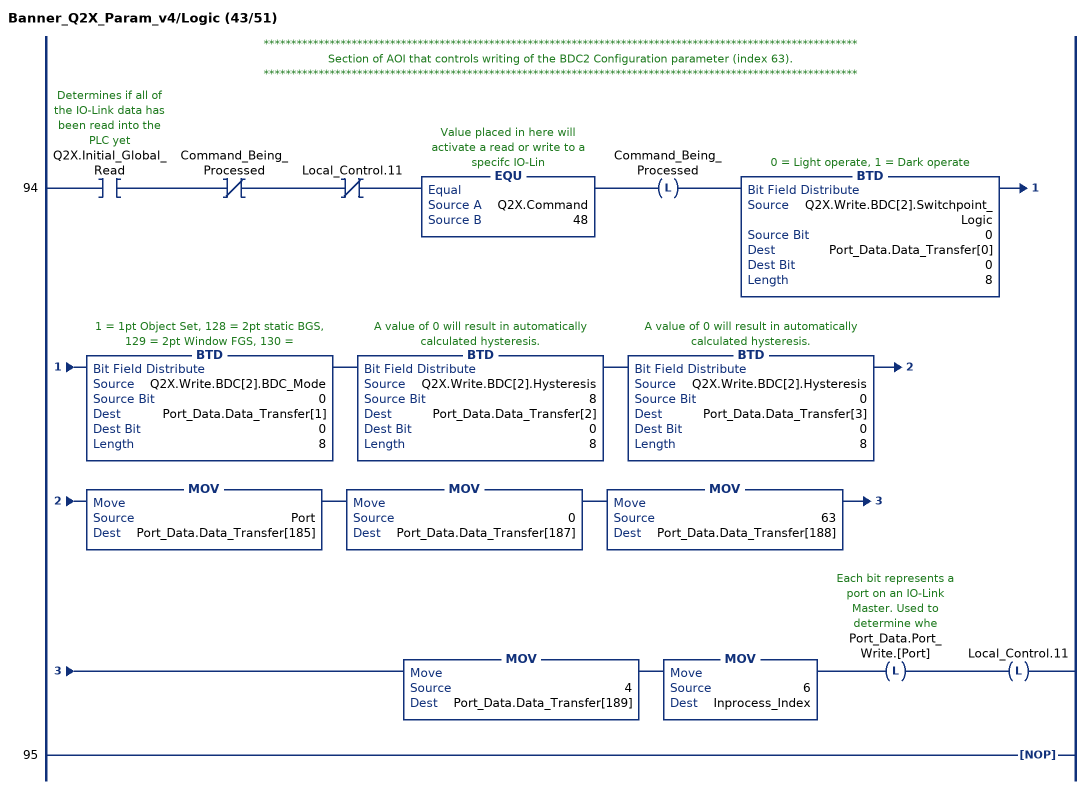
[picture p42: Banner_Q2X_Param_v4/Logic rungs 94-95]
   // ************************************************************************************************************
   // Section of AOI that controls writing of the BDC2 Configuration parameter (index 63).
   // ************************************************************************************************************
   94: XIC(Q2X.Initial_Global_Read)XIO(Command_Being_Processed)XIO(Local_Control.11)EQU(Q2X.Command,48)OTL(Command_Being_Processed)BTD(Q2X.Write.BDC[2].Switchpoint_Logic,0,Port_Data.Data_Transfer[0],0,8)BTD(Q2X.Write.BDC[2].BDC_Mode,0,Port_Data.Data_Transfer[1],0,8)BTD(Q2X.Write.BDC[2].Hysteresis,8,Port_Data.Data_Transfer[2],0,8)BTD(Q2X.Write.BDC[2].Hysteresis,0,Port_Data.Data_Transfer[3],0,8)MOV(Port,Port_Data.Data_Transfer[185])MOV(0,Port_Data.Data_Transfer[187])MOV(63,Port_Data.Data_Transfer[188])MOV(4,Port_Data.Data_Transfer[189])MOV(6,Inprocess_Index)OTL(Port_Data.Port_Write.[Port])OTL(Local_Control.11);
   95: NOP();
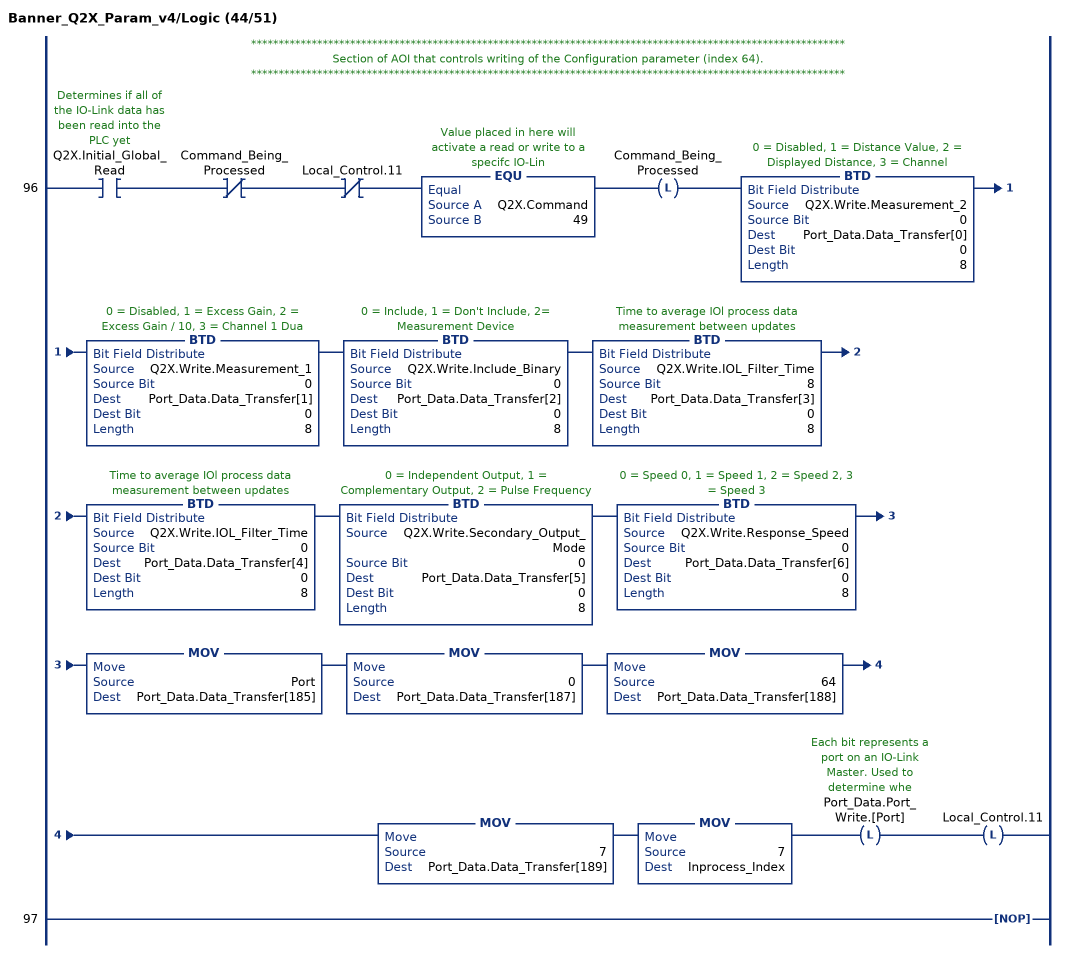
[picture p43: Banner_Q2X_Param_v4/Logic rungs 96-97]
   // ************************************************************************************************************
   // Section of AOI that controls writing of the Configuration parameter (index 64).
   // ************************************************************************************************************
   96: XIC(Q2X.Initial_Global_Read)XIO(Command_Being_Processed)XIO(Local_Control.11)EQU(Q2X.Command,49)OTL(Command_Being_Processed)BTD(Q2X.Write.Measurement_2,0,Port_Data.Data_Transfer[0],0,8)BTD(Q2X.Write.Measurement_1,0,Port_Data.Data_Transfer[1],0,8)BTD(Q2X.Write.Include_Binary,0,Port_Data.Data_Transfer[2],0,8)BTD(Q2X.Write.IOL_Filter_Time,8,Port_Data.Data_Transfer[3],0,8)BTD(Q2X.Write.IOL_Filter_Time,0,Port_Data.Data_Transfer[4],0,8)BTD(Q2X.Write.Secondary_Output_Mode,0,Port_Data.Data_Transfer[5],0,8)BTD(Q2X.Write.Response_Speed,0,Port_Data.Data_Transfer[6],0,8)MOV(Port,Port_Data.Data_Transfer[185])MOV(0,Port_Data.Data_Transfer[187])MOV(64,Port_Data.Data_Transfer[188])MOV(7,Port_Data.Data_Transfer[189])MOV(7,Inprocess_Index)OTL(Port_Data.Port_Write.[Port])OTL(Local_Control.11);
   97: NOP();
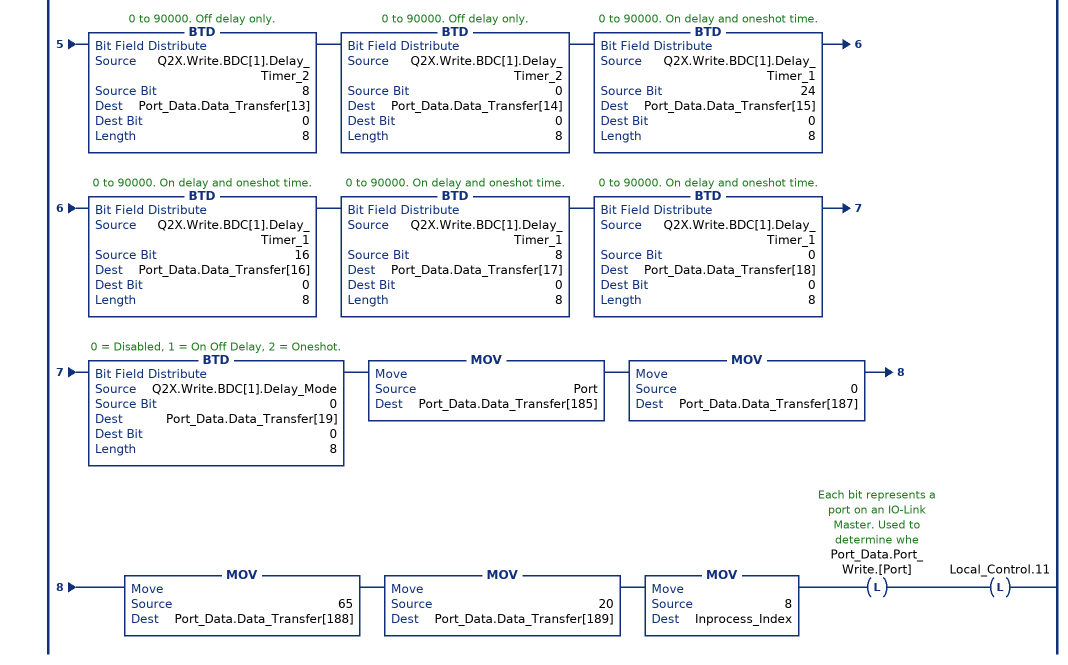
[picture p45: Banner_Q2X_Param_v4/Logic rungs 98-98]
   // ************************************************************************************************************
   // Section of AOI that controls writing of the BDC1 Vendor Specific Configuration parameter (index 65).
   // ************************************************************************************************************
   98: XIC(Q2X.Initial_Global_Read)XIO(Command_Being_Processed)XIO(Local_Control.11)EQU(Q2X.Command,50)OTL(Command_Being_Processed)BTD(Q2X.Write.BDC[1].Auto_Thresholding,0,Port_Data.Data_Transfer[0],0,8)BTD(Q2X.Write.BDC[1].FGS_User_Window_Size,24,Port_Data.Data_Transfer[1],0,8)BTD(Q2X.Write.BDC[1].FGS_User_Window_Size,16,Port_Data.Data_Transfer[2],0,8)BTD(Q2X.Write.BDC[1].FGS_User_Window_Size,8,Port_Data.Data_Transfer[3],0,8)BTD(Q2X.Write.BDC[1].FGS_User_Window_Size,0,Port_Data.Data_Transfer[4],0,8)BTD(Q2X.Write.BDC[1].User_Teach_Offset,24,Port_Data.Data_Transfer[5],0,8)BTD(Q2X.Write.BDC[1].User_Teach_Offset,16,Port_Data.Data_Transfer[6],0,8)BTD(Q2X.Write.BDC[1].User_Teach_Offset,8,Port_Data.Data_Transfer[7],0,8)BTD(Q2X.Write.BDC[1].User_Teach_Offset,0,Port_Data.Data_Transfer[8],0,8)BTD(Q2X.Write.BDC[1].FGS_Window_Size,0,Port_Data.Data_Transfer[9],0,8)BTD(Q2X.Write.BDC[1].Teach_Offset,0,Port_Data.Data_Transfer[10],0,8)BTD(Q2X.Write.BDC[1].Delay_Timer_2,24,Port_Data.Data_Transfer[11],0,8)BTD(Q2X.Write.BDC[1].Delay_Timer_2,16,Port_Data.Data_Transfer[12],0,8)BTD(Q2X.Write.BDC[1].Delay_Timer_2,8,Port_Data.Data_Transfer[13],0,8)BTD(Q2X.Write.BDC[1].Delay_Timer_2,0,Port_Data.Data_Transfer[14],0,8)BTD(Q2X.Write.BDC[1].Delay_Timer_1,24,Port_Data.Data_Transfer[15],0,8)BTD(Q2X.Write.BDC[1].Delay_Timer_1,16,Port_Data.Data_Transfer[16],0,8)BTD(Q2X.Write.BDC[1].Delay_Timer_1,8,Port_Data.Data_Transfer[17],0,8)BTD(Q2X.Write.BDC[1].Delay_Timer_1,0,Port_Data.Data_Transfer[18],0,8)BTD(Q2X.Write.BDC[1].Delay_Mode,0,Port_Data.Data_Transfer[19],0,8)MOV(Port,Port_Data.Data_Transfer[185])MOV(0,Port_Data.Data_Transfer[187])MOV(65,Port_Data.Data_Transfer[188])MOV(20,Port_Data.Data_Transfer[189])MOV(8,Inprocess_Index)OTL(Port_Data.Port_Write.[Port])OTL(Local_Control.11);
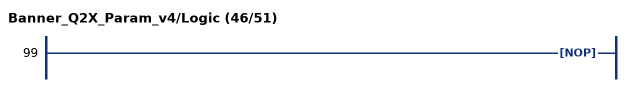
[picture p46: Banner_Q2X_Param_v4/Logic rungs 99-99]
   99: NOP();
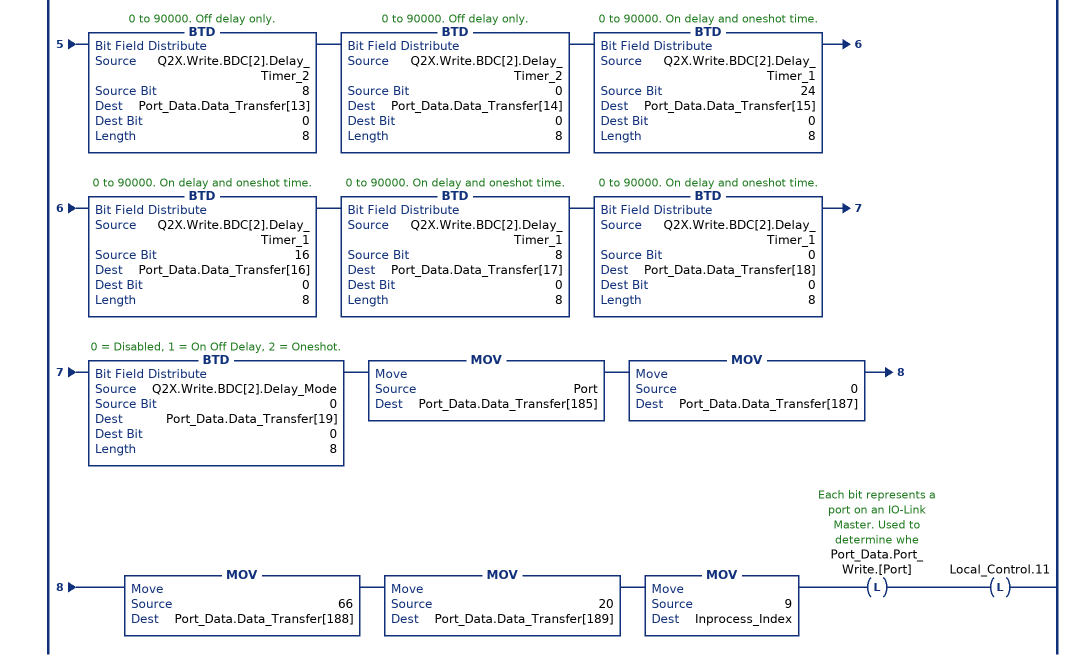
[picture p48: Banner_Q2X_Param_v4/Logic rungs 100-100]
   // ************************************************************************************************************
   // Section of AOI that controls writing of the BDC2 Vendor Specific Configuration parameter (index 66).
   // ************************************************************************************************************
   100: XIC(Q2X.Initial_Global_Read)XIO(Command_Being_Processed)XIO(Local_Control.11)EQU(Q2X.Command,51)OTL(Command_Being_Processed)BTD(Q2X.Write.BDC[2].Auto_Thresholding,0,Port_Data.Data_Transfer[0],0,8)BTD(Q2X.Write.BDC[2].FGS_User_Window_Size,24,Port_Data.Data_Transfer[1],0,8)BTD(Q2X.Write.BDC[2].FGS_User_Window_Size,16,Port_Data.Data_Transfer[2],0,8)BTD(Q2X.Write.BDC[2].FGS_User_Window_Size,8,Port_Data.Data_Transfer[3],0,8)BTD(Q2X.Write.BDC[2].FGS_User_Window_Size,0,Port_Data.Data_Transfer[4],0,8)BTD(Q2X.Write.BDC[2].User_Teach_Offset,24,Port_Data.Data_Transfer[5],0,8)BTD(Q2X.Write.BDC[2].User_Teach_Offset,16,Port_Data.Data_Transfer[6],0,8)BTD(Q2X.Write.BDC[2].User_Teach_Offset,8,Port_Data.Data_Transfer[7],0,8)BTD(Q2X.Write.BDC[2].User_Teach_Offset,0,Port_Data.Data_Transfer[8],0,8)BTD(Q2X.Write.BDC[2].FGS_Window_Size,0,Port_Data.Data_Transfer[9],0,8)BTD(Q2X.Write.BDC[2].Teach_Offset,0,Port_Data.Data_Transfer[10],0,8)BTD(Q2X.Write.BDC[2].Delay_Timer_2,24,Port_Data.Data_Transfer[11],0,8)BTD(Q2X.Write.BDC[2].Delay_Timer_2,16,Port_Data.Data_Transfer[12],0,8)BTD(Q2X.Write.BDC[2].Delay_Timer_2,8,Port_Data.Data_Transfer[13],0,8)BTD(Q2X.Write.BDC[2].Delay_Timer_2,0,Port_Data.Data_Transfer[14],0,8)BTD(Q2X.Write.BDC[2].Delay_Timer_1,24,Port_Data.Data_Transfer[15],0,8)BTD(Q2X.Write.BDC[2].Delay_Timer_1,16,Port_Data.Data_Transfer[16],0,8)BTD(Q2X.Write.BDC[2].Delay_Timer_1,8,Port_Data.Data_Transfer[17],0,8)BTD(Q2X.Write.BDC[2].Delay_Timer_1,0,Port_Data.Data_Transfer[18],0,8)BTD(Q2X.Write.BDC[2].Delay_Mode,0,Port_Data.Data_Transfer[19],0,8)MOV(Port,Port_Data.Data_Transfer[185])MOV(0,Port_Data.Data_Transfer[187])MOV(66,Port_Data.Data_Transfer[188])MOV(20,Port_Data.Data_Transfer[189])MOV(9,Inprocess_Index)OTL(Port_Data.Port_Write.[Port])OTL(Local_Control.11);
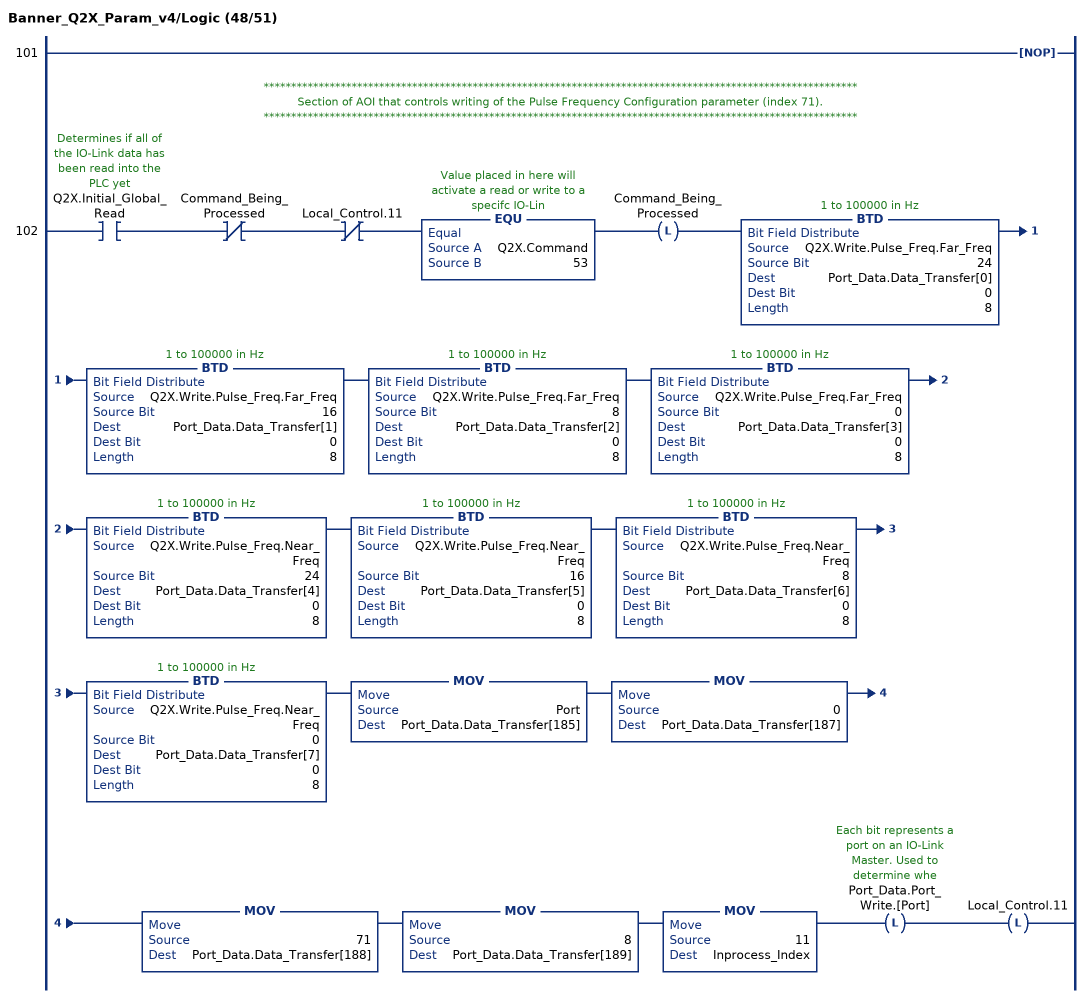
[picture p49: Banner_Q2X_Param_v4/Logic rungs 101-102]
   101: NOP();
   // ************************************************************************************************************
   // Section of AOI that controls writing of the Pulse Frequency Configuration parameter (index 71).
   // ************************************************************************************************************
   102: XIC(Q2X.Initial_Global_Read)XIO(Command_Being_Processed)XIO(Local_Control.11)EQU(Q2X.Command,53)OTL(Command_Being_Processed)BTD(Q2X.Write.Pulse_Freq.Far_Freq,24,Port_Data.Data_Transfer[0],0,8)BTD(Q2X.Write.Pulse_Freq.Far_Freq,16,Port_Data.Data_Transfer[1],0,8)BTD(Q2X.Write.Pulse_Freq.Far_Freq,8,Port_Data.Data_Transfer[2],0,8)BTD(Q2X.Write.Pulse_Freq.Far_Freq,0,Port_Data.Data_Transfer[3],0,8)BTD(Q2X.Write.Pulse_Freq.Near_Freq,24,Port_Data.Data_Transfer[4],0,8)BTD(Q2X.Write.Pulse_Freq.Near_Freq,16,Port_Data.Data_Transfer[5],0,8)BTD(Q2X.Write.Pulse_Freq.Near_Freq,8,Port_Data.Data_Transfer[6],0,8)BTD(Q2X.Write.Pulse_Freq.Near_Freq,0,Port_Data.Data_Transfer[7],0,8)MOV(Port,Port_Data.Data_Transfer[185])MOV(0,Port_Data.Data_Transfer[187])MOV(71,Port_Data.Data_Transfer[188])MOV(8,Port_Data.Data_Transfer[189])MOV(11,Inprocess_Index)OTL(Port_Data.Port_Write.[Port])OTL(Local_Control.11);
